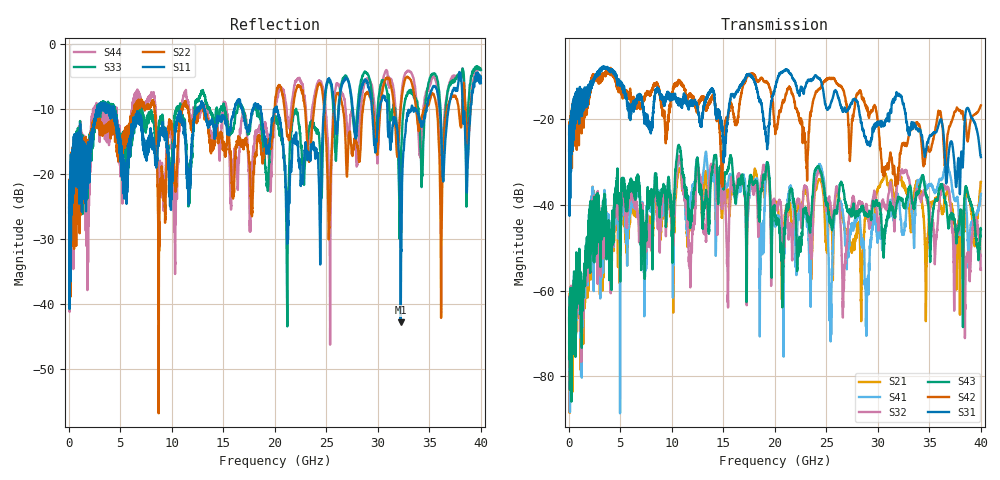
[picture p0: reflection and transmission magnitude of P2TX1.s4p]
!Agilent Technologies,N5245A,MY49151084,A.09.20.08
!Agilent N5245A: A.09.20.08
!Date: Thursday, March 01, 2012 11:45:11
!Correction: S11(Full 4 Port(1,2,3,4))
!S12(Full 4 Port(1,2,3,4))
!S13(Full 4 Port(1,2,3,4))
!S14(Full 4 Port(1,2,3,4))
!S21(Full 4 Port(1,2,3,4))
!S22(Full 4 Port(1,2,3,4))
!S23(Full 4 Port(1,2,3,4))
!S24(Full 4 Port(1,2,3,4))
!S31(Full 4 Port(1,2,3,4))
!S32(Full 4 Port(1,2,3,4))
!S33(Full 4 Port(1,2,3,4))
!S34(Full 4 Port(1,2,3,4))
!S41(Full 4 Port(1,2,3,4))
!S42(Full 4 Port(1,2,3,4))
!S43(Full 4 Port(1,2,3,4))
!S44(Full 4 Port(1,2,3,4))
!S4P File: Measurements: <S11,S12,S13,S14>,
!<S21,S22,S23,S24>,
!<S31,S32,S33,S34>,
!<S41,S42,S43,S44>:
# Hz S  dB  R 50
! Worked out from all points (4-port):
!   3996 points, 50 MHz to 40 GHz, reference 50 ohm
!   strongest paths, dB at 50 MHz, 10.04 GHz, 20.03 GHz, 30.02 GHz, 40 GHz:
!     S31: -27.3, -14.3, -12.5, -20.9, -28.8
!     S42: -23.5, -14.0, -22.6, -21.2, -16.8
!     S43: -66.4, -47.4, -42.7, -40.0, -45.6
!     S32: -64.6, -47.0, -40.0, -44.0, -55.1
!     S41: -71.9, -44.9, -44.6, -47.1, -37.4
!     S21: -75.7, -46.1, -39.9, -36.0, -34.6
!   lowest |S11| = -42.8 dB at 32.22 GHz (marker M1), VSWR 1.01, Z = 49.7 - j0.669 ohm
!   |S11| at or under -10 dB: 4.38 GHz to 12.49 GHz (8.105 GHz wide, 96.1 % of centre); 13.15 GHz to 16.1 GHz (2.948 GHz wide, 20.2 % of centre); 20.21 GHz to 24.77 GHz (4.566 GHz wide, 20.3 % of centre)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
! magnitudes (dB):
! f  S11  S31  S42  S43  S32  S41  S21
! 50 MHz  -25.1  -27.3  -23.5  -66.4  -64.6  -71.9  -75.7
! 2.42 GHz  -13.7  -11.1  -10.0  -44.9  -40.8  -42.9  -39.3
! 10.72 GHz  -10.7  -16.8  -10.9  -26.2  -28.6  -29.5  -31.7
! 11.79 GHz  -22.3  -16.6  -14.5  -45.4  -56.8  -39.2  -42.5
! 26.69 GHz  -5.8  -17.9  -13.6  -37.1  -59.4  -43.9  -44.2
! 32.22 GHz  -42.8  -14.4  -27.6  -38.5  -32.4  -43.4  -34.1
! 40 GHz  -6.0  -28.8  -16.8  -45.6  -55.1  -37.4  -34.6
